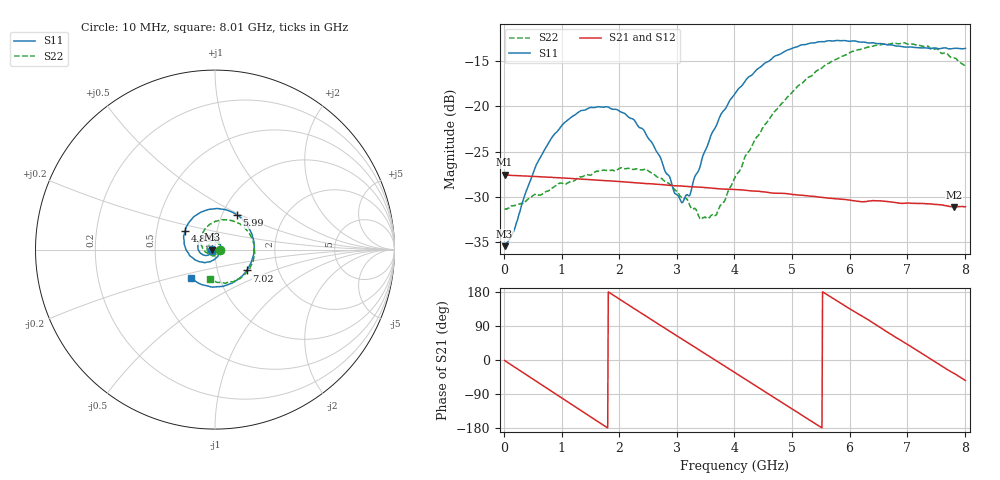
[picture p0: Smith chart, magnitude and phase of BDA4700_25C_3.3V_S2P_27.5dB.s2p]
!Agilent Technologies,E5071B,MY42404982,A.09.10
!Date: Mon Oct 20 18:14:38 2025
!Data & Calibration Information:
!Freq	S11:SOLT2(ON)	S21:SOLT2(ON)	S12:SOLT2(ON)	S22:SOLT2(ON)
# Hz S RI R 50
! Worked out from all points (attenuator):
!   801 points, 10 MHz to 8.01 GHz, reference 50 ohm
!   highest |S21| = -27.56 dB at 10 MHz (marker M1); lowest = -31.1 dB at 7.81 GHz (marker M2)
!   lowest |S11| = -35.4 dB at 10 MHz (marker M3), VSWR 1.03, Z = 48.3 - j0.0991 ohm
!   |S11| at or under -10 dB: start of sweep to end of sweep
!   |S22| runs from -32.5 to -13.0 dB; largest |S21 - S12| = 0.00046
!   S11 on the Smith chart (normalised r, x): 10 MHz: 0.97, -0.00; 4.83 GHz: 0.70, +0.15; 5.99 GHz: 1.17, +0.48; 7.02 GHz: 1.38, -0.34; 8.01 GHz: 0.73, -0.25
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1e7  -0.0169 -0.00102  0.0419 -0.00092  0.0418 -0.000929  0.0272 -0.00083
1.6e8  -0.0177 -0.00972  0.0399 -0.0118  0.0398 -0.0117  0.0273 -0.00772
5.3e8  -0.0344 -0.0289  0.0244 -0.033  0.0244 -0.033  0.0168 -0.0281
7.1e8  -0.0479 -0.0326  0.0129 -0.0386  0.013 -0.0386  0.00542 -0.0332
1.35e9  -0.0946 0.00383  -0.028 -0.028  -0.028 -0.028  -0.0365 -0.0183
2.08e9  -0.054 0.0741  -0.0342 0.0172  -0.0342 0.0172  -0.0302 0.0338
2.42e9  -0.0102 0.0736  -0.0188 0.0325  -0.0188 0.0325  -0.00519 0.0445
2.68e9  0.0178 0.0514  -0.00308 0.037  -0.00314 0.0369  0.0129 0.0383
2.96e9  0.0302 0.014  0.0138 0.0338  0.0138 0.0337  0.0259 0.0233
3.11e9  0.0285 -0.00869  0.0217 0.0291  0.0216 0.0291  0.0289 0.011
3.23e9  0.0219 -0.0242  0.0269 0.024  0.0269 0.024  0.028 0.00286
3.55e9  -0.0149 -0.0611  0.0348 0.00672  0.0349 0.00667  0.0132 -0.0202
3.7e9  -0.0406 -0.0689  0.0351 -0.00218  0.0352 -0.00222  0.000421 -0.0259
4.01e9  -0.0995 -0.0623  0.0291 -0.0191  0.029 -0.0191  -0.031 -0.026
4.83e9  -0.1671 0.1033  -0.0127 -0.0306  -0.0125 -0.0306  -0.0766 0.0708
5.35e9  -0.0728 0.2106  -0.0305 -0.00944  -0.0304 -0.00964  -0.0159 0.1467
5.99e9  0.1201 0.1936  -0.022 0.021  -0.0221 0.0209  0.1285 0.1479
6.68e9  0.2173 -0.00568  0.00949 0.0282  0.00962 0.0283  0.2194 0.000762
7.02e9  0.1774 -0.1161  0.0225 0.0187  0.0226 0.0186  0.2001 -0.0906
7.45e9  0.0544 -0.2018  0.0288 -0.00069  0.0289 -0.000791  0.1131 -0.1706
7.81e9  -0.0717 -0.195  0.0228 -0.0161  0.0228 -0.0162  0.0176 -0.1838
8.01e9  -0.1318 -0.161  0.0164 -0.0227  0.0165 -0.0227  -0.0301 -0.1634
